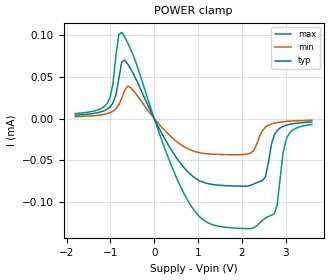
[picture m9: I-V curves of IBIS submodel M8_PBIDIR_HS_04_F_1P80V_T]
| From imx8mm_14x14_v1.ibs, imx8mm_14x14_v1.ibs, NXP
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| Submodel
[Submodel]  M8_PBIDIR_HS_04_F_1P80V_T
Submodel_type Dynamic_clamp
[POWER Clamp]
| Voltage   I(typ)   I(min)   I(max)
-1.8V     4.081uA    2.137uA    5.96uA
-1.076V   11.15uA    5.88uA     18.05uA
-941.4mV  18.7uA     8.834uA    41.7uA
-874.1mV  28.3uA     11.67uA    75.87uA
-739.7mV  68.27uA    24.59uA    103.5uA
-537.9mV  59.8uA     37.23uA    83.25uA
806.9mV   -66.08uA   -37.25uA   -102.1uA
2.002V    -81.28uA   -43.4uA    -132uA
2.54V     -69.93uA   -10.28uA   -119.6uA
2.741V    -19.89uA   -5.491uA   -114.3uA
3.01V     -7.987uA   -3.507uA   -25.3uA
3.6V      -4.108uA   -2.027uA   -7.198uA
